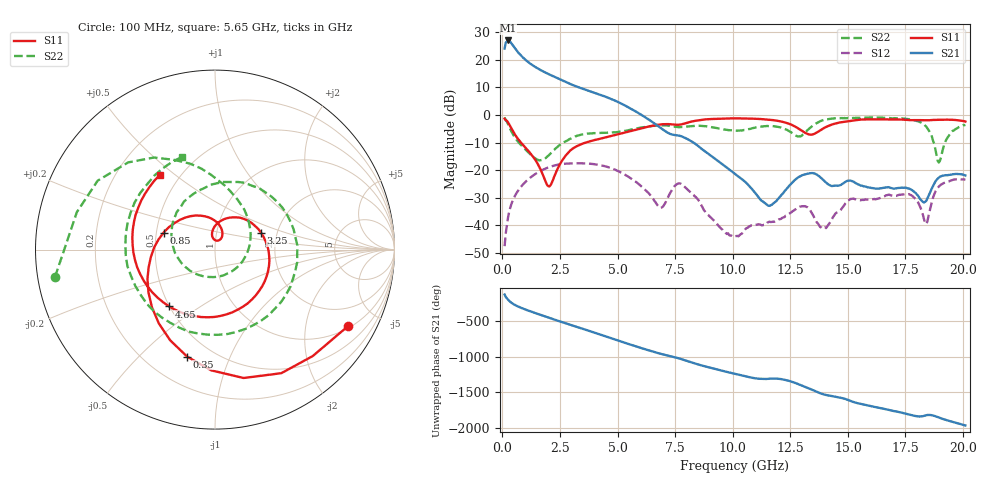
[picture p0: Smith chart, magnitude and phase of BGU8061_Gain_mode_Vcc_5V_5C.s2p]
# GHZ S DB R 50
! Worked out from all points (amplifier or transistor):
!   401 points, 100 MHz to 20.1 GHz, reference 50 ohm
!   highest |S21| = 27.0 dB at 250 MHz (marker M1)
!   |S21| within 3 dB of that: start of sweep to 565.5 MHz
!   unconditionally stable (mu >= 1): start of sweep to end of sweep
!   at 3.4 GHz: K = 1.23, MAG = 10.8 dB, |S12| = -17.5 dB
!   at 10.1 GHz: K = 166.12, MAG = -13.9 dB, |S12| = -44.0 dB
!   at 20.1 GHz: K = 21.49, MAG = -15.6 dB, |S12| = -23.4 dB
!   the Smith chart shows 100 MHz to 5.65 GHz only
!   S11 on the Smith chart (normalised r, x): 100 MHz: 1.08, -3.41; 350 MHz: 0.37, -0.71; 850 MHz: 0.55, +0.11; 3.25 GHz: 1.65, +0.33; 4.65 GHz: 0.50, -0.38; 5.65 GHz: 0.39, +0.44
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0.1  -1.37 -30.1  24.09 -127.4  -47.57 120.5  -0.88 -170.3
0.25  -2.70 -77.5  27.02 159.9  -37.11 89.4  -3.27 134.9
0.35  -4.21 -104.6  26.46 128.5  -33.46 71.5  -5.21 114.4
0.45  -5.73 -127.2  25.35 104.7  -31.06 56.4  -6.82 99.3
0.6  -7.74 -156.6  23.63 77.0  -28.54 36.2  -8.83 81.6
0.85  -10.42 161.7  21.22 41.1  -25.64 6.6  -11.16 53.9
1.3  -14.74 101.1  18.11 -13.4  -22.17 -43.6  -14.87 -5.7
1.75  -21.49 61.8  15.89 -63.6  -19.91 -93.3  -16.29 -92.3
2.5  -17.84 91.2  12.94 -145.8  -17.89 -176.8  -10.87 142.2
3.25  -11.26 20.0  10.23 135.3  -17.53 101.5  -7.50 54.3
3.45  -10.51 -0.8  9.63 114.4  -17.53 80.1  -7.07 31.3
4.1  -8.92 -69.3  7.75 45.6  -17.96 10.1  -6.58 -44.1
4.65  -7.80 -128.9  6.06 -13.7  -19.06 -50.3  -6.41 -114.3
5.65  -5.72 126.5  1.96 -121.6  -23.37 -154.9  -5.21 109.6
6.8  -3.51 21.9  -4.27 124.5  -33.37 125.1  -3.79 -28.3
8.35  -2.15 -86.9  -10.32 -16.8  -29.46 -39.9  -3.93 177.9
10.1  -1.22 162.4  -21.39 -164.4  -43.96 123.8  -5.66 -24.5
12.4  -3.05 19.0  -26.21 100.6  -36.07 -98.3  -5.61 121.0
13.45  -7.10 -132.3  -21.07 -29.1  -35.83 70.1  -4.05 110.4
14.7  -2.64 80.4  -25.36 -141.8  -34.33 -136.3  -1.18 46.2
16.8  -1.64 -23.5  -26.24 45.2  -28.93 33.7  -1.10 -42.7
20.1  -2.38 -162.3  -21.93 -171.0  -23.41 -139.9  -3.59 -118.9
